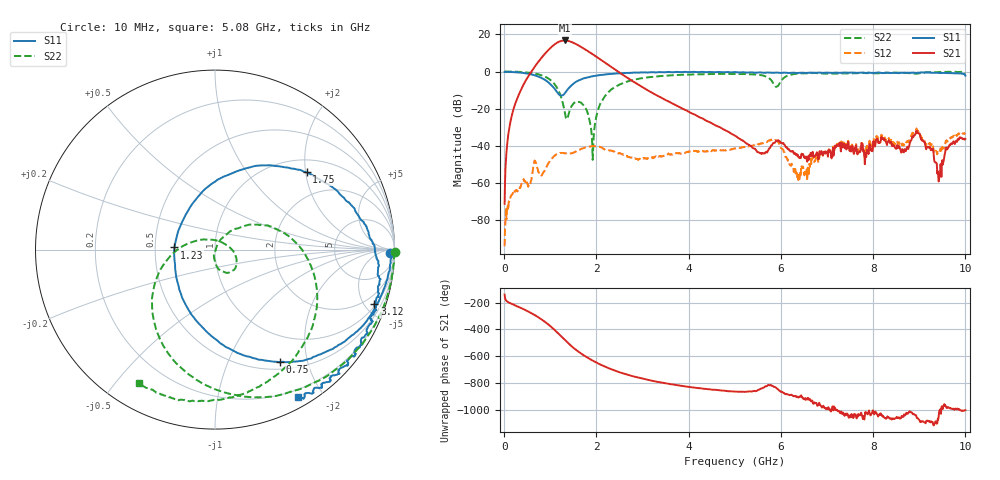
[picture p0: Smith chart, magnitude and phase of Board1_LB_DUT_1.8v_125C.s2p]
! Created Tue May 27 17:11:51 2025
# hz S ma R 50
! 2 Port Network Data from SP1.SP block
! freq  magS11  angS11  magS21  angS21  magS12  angS12  magS22  angS22
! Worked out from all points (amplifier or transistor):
!   1000 points, 10 MHz to 10 GHz, reference 50 ohm
!   highest |S21| = 16.8 dB at 1.31 GHz (marker M1)
!   |S21| within 3 dB of that: 1.05 GHz to 1.635 GHz (584.7 MHz wide, 43.6 % of centre)
!   unconditionally stable (mu >= 1): 15.82 MHz to 49.85 MHz; 50.09 MHz to end of sweep
!   at 1.67 GHz: K = 8.35, MAG = 15.3 dB, |S12| = -41.9 dB
!   at 5.01 GHz: K = 54.52, MAG = -17.0 dB, |S12| = -41.4 dB
!   at 10 GHz: K = 95.89, MAG = -24.2 dB, |S12| = -33.6 dB
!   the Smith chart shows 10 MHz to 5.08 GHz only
!   S11 on the Smith chart (normalised r, x): 10 MHz: 51, -41; 750 MHz: 0.59, -1.57; 1.23 GHz: 0.63, +0.02; 1.75 GHz: 1.30, +2.02; 3.12 GHz: 1.14, -5.79; 5.08 GHz: 0.12, -1.71
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1e7  0.9765 -1.1  0.0002665 -139.1  1.919e-05 177.9  1.003 -0.9
2e8  0.9645 -13.7  0.09366 146.0  0.0005809 74.0  0.9923 -17.9
7.5e8  0.7238 -60.1  1.883 48.4  0.001916 64.2  0.8367 -78.4
9.1e8  0.5661 -80.6  3.272 10.0  0.002534 107.8  0.7009 -103.3
1.05e9  0.3961 -107.3  4.881 -30.1  0.004724 97.5  0.5228 -130.6
1.14e9  0.2864 -135.1  5.916 -58.9  0.005816 84.0  0.3744 -152.1
1.23e9  0.226 177.0  6.658 -89.7  0.006267 70.3  0.2122 -179.4
1.31e9  0.2532 130.3  6.895 -117.3  0.006181 62.1  0.08542 138.5
1.47e9  0.4324 78.1  6.206 -168.4  0.006227 58.3  0.1204 -17.3
1.68e9  0.6207 46.7  4.511 136.6  0.008218 50.3  0.1391 -65.8
1.75e9  0.6674 40.1  3.994 120.9  0.00879 44.1  0.1111 -80.0
1.92e9  0.7471 27.1  2.918 86.4  0.009563 27.1  0.004107 -34.8
2.13e9  0.8112 15.1  1.942 49.9  0.008601 3.9  0.1682 44.1
2.51e9  0.8928 -0.8  0.9228 -1.8  0.006225 -7.3  0.4492 5.3
3.12e9  0.9383 -18.9  0.3056 -57.5  0.004567 9.9  0.6963 -39.4
3.34e9  0.9555 -24.4  0.2161 -72.9  0.005187 8.3  0.7427 -52.5
5.01e9  0.9665 -59.4  0.0183 -145.0  0.008486 -10.1  0.8599 -117.0
5.08e9  0.9429 -60.5  0.01591 -146.4  0.008761 -10.8  0.8541 -119.5
6.67e9  0.9292 -90.1  0.005626 146.7  0.003751 138.7  0.9073 -150.8
8.34e9  0.9114 -135.2  0.01392 20.4  0.01599 31.8  0.9226 172.6
9.43e9  0.9144 -166.3  0.001249 61.7  0.006466 60.9  0.9653 168.5
1e10  0.7762 176.0  0.01508 75.8  0.02079 67.9  0.9219 168.2
